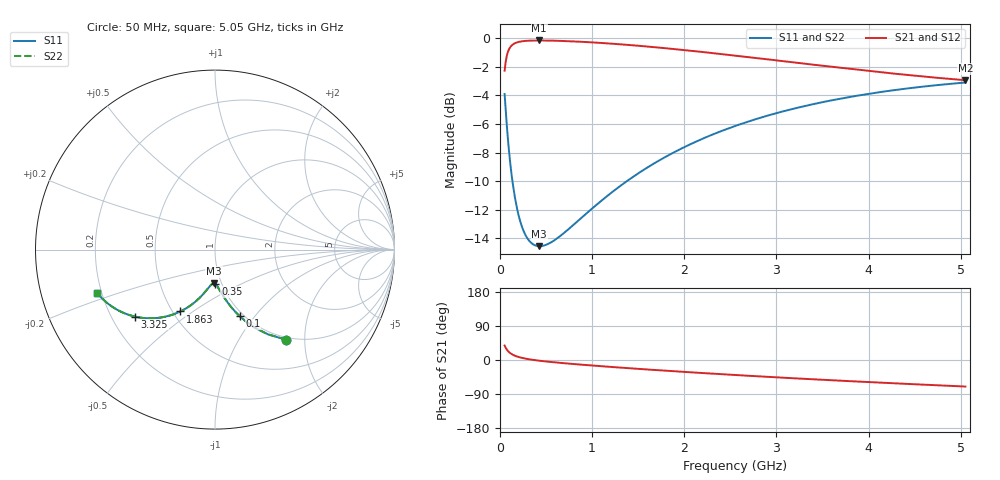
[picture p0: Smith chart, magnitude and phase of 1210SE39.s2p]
! AVX Thin Film Operation		Date: August 2001
! Description: Accu-P® Series, Thin Film, SMD, RF Capacitor
! Part Number: 12101J390FBT
! 50 MHz  -  5.05 GHz
! Serial Measurements
# mhz S db R 50
!	S11		S21		S12		S22
!	dB	Phase	dB	Phase	dB	Phase	dB	Phase
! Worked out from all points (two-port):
!   401 points, 50 MHz to 5.05 GHz, reference 50 ohm
!   highest |S21| = -0.16 dB at 425 MHz (marker M1); lowest = -2.9 dB at 5.05 GHz (marker M2)
!   |S21| within 3 dB of the highest: start of sweep to end of sweep
!   lowest |S11| = -14.6 dB at 425 MHz (marker M3), VSWR 1.46, Z = 46.1 - j17.9 ohm
!   |S11| at or under -10 dB: 134.9 MHz to 1.377 GHz (1.242 GHz wide, 164 % of centre)
!   |S22| runs from -14.6 to -3.1 dB; largest |S21 - S12| = 8.9e-05
!   S11 on the Smith chart (normalised r, x): 50 MHz: 0.96, -1.62; 100 MHz: 0.96, -0.84; 350 MHz: 0.93, -0.37; 1.863 GHz: 0.55, -0.45; 3.325 GHz: 0.30, -0.34; 5.05 GHz: 0.18, -0.17
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50  -3.90 -51.8  -2.27 38.2  -2.27 38.2  -3.90 -51.8
75  -6.20 -62.9  -1.20 27.1  -1.20 27.1  -6.20 -62.9
87.5  -7.17 -66.6  -0.93 23.4  -0.93 23.4  -7.17 -66.6
100  -8.05 -69.6  -0.74 20.4  -0.74 20.4  -8.05 -69.6
112.5  -8.82 -72.1  -0.61 17.9  -0.61 17.9  -8.82 -72.1
137.5  -10.13 -75.9  -0.45 14.1  -0.45 14.1  -10.13 -75.9
162.5  -11.17 -78.7  -0.35 11.2  -0.35 11.2  -11.17 -78.7
200  -12.34 -81.9  -0.26 8.0  -0.26 8.0  -12.34 -81.9
262.5  -13.59 -85.6  -0.20 4.3  -0.20 4.3  -13.59 -85.6
350  -14.38 -89.3  -0.16 0.6  -0.16 0.6  -14.38 -89.3
425  -14.55 -91.7  -0.16 -1.8  -0.16 -1.8  -14.55 -91.7
587.5  -14.15 -96.0  -0.17 -6.1  -0.17 -6.1  -14.15 -96.0
887.5  -12.55 -102.3  -0.25 -12.4  -0.25 -12.4  -12.55 -102.4
1300  -10.36 -109.9  -0.42 -20.0  -0.42 -20.0  -10.36 -109.9
1725  -8.56 -117.0  -0.66 -27.1  -0.66 -27.1  -8.56 -117.0
1862.5  -8.07 -119.2  -0.74 -29.3  -0.74 -29.3  -8.07 -119.2
2200  -7.03 -124.4  -0.96 -34.5  -0.96 -34.5  -7.03 -124.4
2550  -6.14 -129.6  -1.21 -39.6  -1.21 -39.6  -6.14 -129.6
3325  -4.72 -140.0  -1.80 -50.0  -1.80 -50.0  -4.72 -140.0
3387.5  -4.63 -140.8  -1.84 -50.8  -1.84 -50.8  -4.63 -140.8
4225  -3.68 -150.9  -2.44 -60.9  -2.44 -60.9  -3.68 -150.9
5050  -3.10 -160.0  -2.94 -70.0  -2.94 -70.0  -3.10 -160.0
